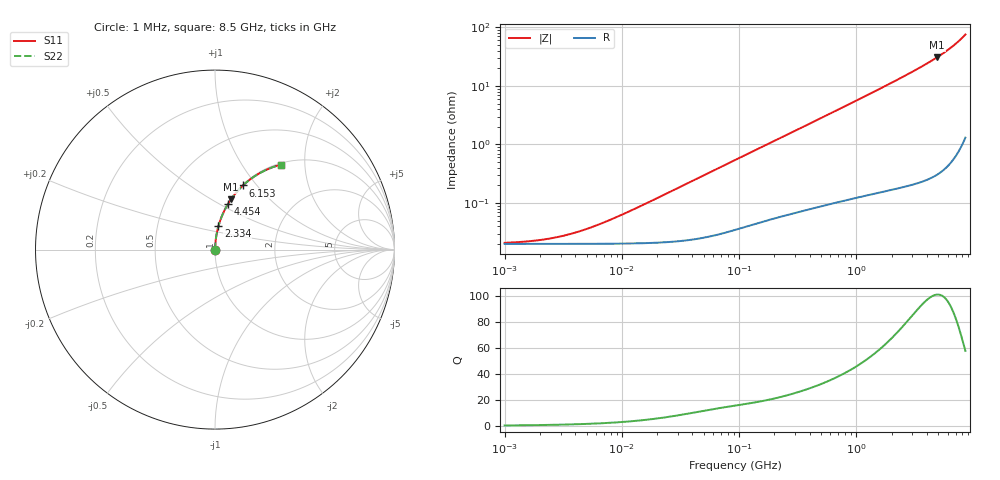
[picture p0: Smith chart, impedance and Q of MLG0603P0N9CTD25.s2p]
! S-Parameter Data Generated by TDK Corporation
! Copyright(C) 2025 TDK Corporation.
! All Rights Reserved.
! TDK P/N: MLG0603P0N9CTD25 (SMD / SMT Inductor (Coil))
! Property: L=0.9nH at 500MHz
! Size(LxWxT): 0.6x0.3x0.3mm
! Model Type: s2p (Touchstone File Format Version 1.0)
! Frequency: DC=Yes Start=1MHz Stop=8500MHz 198points Log-sweep
! Model Generated on Feb. 6, 2025
! Terms and conditions regarding TDK Simulation Models:
! 1)This simulation model is being provided solely for informational
!  purposes. Please refer to the specifications of the products in
!  terms of detailed characteristics of such products.
! 2)In no event shall TDK Corporation of any of its subsidiaries be
!  liable for any loss or damage arising, directly or indirectly,
!  from any information contained in this simulation model, including,
!  but not limited to loss or damages arising from any inaccuracies,
!  omissions or errors in connection with such information.
! 3)Any and all copyrights on this simulation model are owned by
!  TDK Corporation.  Duplication or redistribution of this simulation
!  model without prior written permission from TDK Corporation
!  is prohibited.
! 4)This simulation model is subject to any modification or change
!  without any prior notice.
! 5)Neither TDK Corporation nor any of its subsidiaries shall make any
!  warranty, express or implied, including but not limited to the
!  correctness, implied warranties of merchantability and fitness for
!  a particular purpose with respect to this simulation models.
! 6)The use of this simulation model shall be deemed to have consented
!  to the terms and conditions hereof.
! Port Assignments:
!  1 ---@@@--- 2
! Applicable Conditions:
!  Temperature = 25 degC
!  DC Bias Current = 0 A
!  Small Signal Operation
# Hz S MA R 50
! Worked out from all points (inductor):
!   197 points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, 1 MHz to 8.5 GHz, reference 50 ohm
!   read as one part in series: L = 951 pH near 10.53 MHz
!   highest Q = 101 at 4.885 GHz (marker M1), where L = 1.01 nH
!   S11 on the Smith chart (normalised r, x): 1 MHz: 1.00, +0.00; 2.334 GHz: 1.00, +0.27; 4.454 GHz: 1.01, +0.55; 6.153 GHz: 1.01, +0.85; 8.5 GHz: 1.03, +1.51
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1000000  0.0002087 16.6  0.9998 -0.0  0.9998 -0.0  0.0002087 16.6
1586648  0.0002214 25.4  0.9998 -0.0  0.9998 -0.0  0.0002214 25.4
2295435  0.0002426 34.4  0.9998 -0.0  0.9998 -0.0  0.0002426 34.4
3320851  0.0002819 44.7  0.9998 -0.0  0.9998 -0.0  0.0002819 44.7
4587603  0.0003396 53.8  0.9998 -0.0  0.9998 -0.0  0.0003396 53.8
6337562  0.0004287 62.0  0.9998 -0.0  0.9998 -0.0  0.0004287 62.0
8755050  0.0005606 68.9  0.9998 -0.0  0.9998 -0.0  0.0005606 68.9
2.10461e7  0.001273 80.4  0.9998 -0.1  0.9998 -0.1  0.001273 80.4
9.219544e7  0.005422 86.0  0.9996 -0.3  0.9996 -0.3  0.005422 86.0
4.229561e8  0.02397 86.7  0.9989 -1.4  0.9989 -1.4  0.02397 86.7
1.016736e9  0.05703 85.5  0.9971 -3.3  0.9971 -3.3  0.05703 85.5
1.940355e9  0.1093 82.9  0.9924 -6.3  0.9924 -6.3  0.1093 82.9
2.333852e9  0.132 81.6  0.9895 -7.6  0.9895 -7.6  0.132 81.6
3.224109e9  0.1854 78.7  0.9806 -10.7  0.9806 -10.7  0.1854 78.7
4.453958e9  0.2648 74.1  0.9617 -15.4  0.9617 -15.4  0.2648 74.1
4.884749e9  0.2945 72.3  0.9527 -17.1  0.9527 -17.1  0.2945 72.3
5.610304e9  0.3475 69.1  0.9342 -20.3  0.9342 -20.3  0.3475 69.1
6.152938e9  0.3896 66.5  0.9169 -22.9  0.9169 -22.9  0.3896 66.5
6.748056e9  0.4384 63.3  0.8937 -26.0  0.8937 -26.0  0.4384 63.3
7.400733e9  0.4954 59.6  0.8623 -29.7  0.8623 -29.7  0.4954 59.6
8.116539e9  0.5617 54.9  0.8187 -34.2  0.8187 -34.2  0.5617 54.9
8.5e9  0.5987 52.2  0.7907 -36.8  0.7907 -36.8  0.5987 52.2
